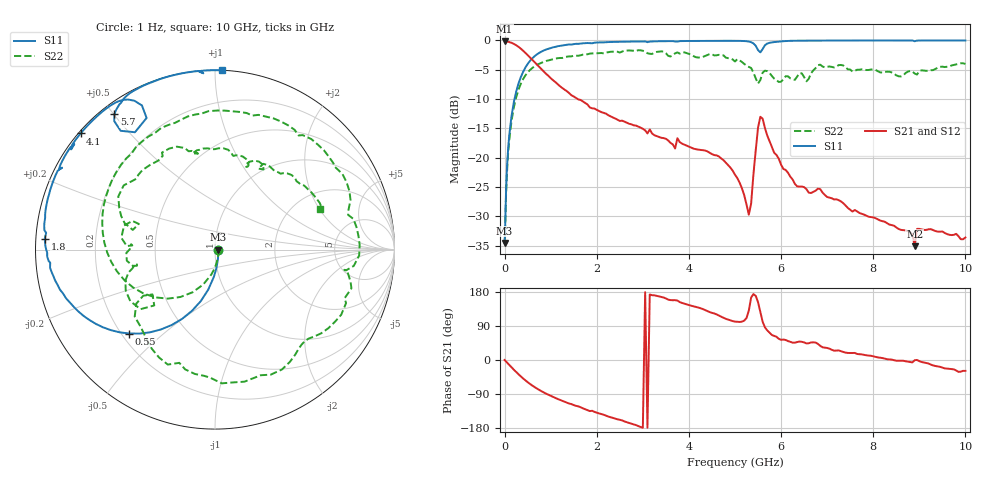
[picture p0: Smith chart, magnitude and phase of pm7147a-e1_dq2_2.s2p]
# GHz S DB R 50
! S-Parameters data
! Freq  dbS11  angS11  dbS21  angS21  dbS12  angS12  dbS22  angS22
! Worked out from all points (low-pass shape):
!   279 points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, 1 Hz to 10 GHz, reference 50 ohm
!   highest |S21| = -0.16 dB at 1.6 Hz (marker M1); lowest = -35.1 dB at 8.9 GHz (marker M2)
!   |S21| within 3 dB of the highest: start of sweep to 582.4 MHz
!   lowest |S11| = -34.5 dB at 25.1 Hz (marker M3), VSWR 1.04, Z = 51.9 - j3.19e-06 ohm
!   |S11| at or under -10 dB: start of sweep to 215 MHz
!   |S22| runs from -34.5 to -1.7 dB; largest |S21 - S12| = 3.8e-13
!   S11 on the Smith chart (normalised r, x): 1 Hz: 1.04, -0.00; 550 MHz: 0.23, -0.39; 1.8 GHz: 0.03, +0.03; 4.1 GHz: 0.01, +0.37; 5.7 GHz: 0.04, +0.50; 10 GHz: 0.00, +1.04
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1e-09  -34.54 -0.0  -0.16 -0.0  -0.16 -0.0  -34.54 -0.0
1.6e-09  -34.54 -0.0  -0.16 -0.0  -0.16 -0.0  -34.54 -0.0
2.51e-08  -34.54 -0.0  -0.16 -0.0  -0.16 -0.0  -34.54 -0.0
0.06309573  -20.10 -85.0  -0.21 -8.2  -0.21 -8.2  -20.88 -88.0
0.15  -12.87 -99.7  -0.41 -19.3  -0.41 -19.3  -13.71 -108.7
0.55  -3.49 -135.6  -2.90 -63.1  -2.90 -63.1  -5.05 -167.5
1  -1.29 -160.1  -6.43 -94.7  -6.43 -94.7  -3.29 149.7
1.7  -0.49 178.7  -10.40 -127.6  -10.40 -127.6  -2.42 101.6
1.8  -0.44 176.3  -10.93 -132.5  -10.93 -132.5  -2.36 95.4
2.55  -0.23 161.8  -13.69 -159.4  -13.69 -159.4  -1.90 52.6
3.35  -0.14 149.4  -16.44 167.9  -16.44 167.9  -1.91 5.4
4.1  -0.09 139.2  -18.44 141.7  -18.44 141.7  -2.68 -41.3
4.65  -0.07 132.0  -19.78 117.2  -19.78 117.2  -2.45 -77.4
5.05  -0.07 126.4  -23.46 100.9  -23.46 100.9  -3.19 -112.3
5.3  -0.19 121.5  -29.72 130.6  -29.72 130.6  -4.52 -134.8
5.55  -2.03 124.3  -13.01 126.9  -13.01 126.9  -6.75 -137.4
5.7  -0.53 126.5  -16.22 78.0  -16.22 78.0  -5.23 -155.3
6.7  -0.03 113.1  -25.81 46.6  -25.81 46.6  -5.11 160.3
7.35  -0.01 107.0  -27.76 21.2  -27.76 21.2  -4.27 110.3
8.35  -0.01 98.9  -31.39 1.5  -31.39 1.5  -5.34 73.3
8.9  -0.14 93.8  -35.08 -0.6  -35.08 -0.6  -5.64 58.8
10  -0.00 87.7  -33.60 -28.7  -33.60 -28.7  -4.01 21.2
